FUNCTION "Ramp_down_folgen" : VOID
TITLE =
AUTHOR : 'Kleißler'
VERSION : 0.1

BEGIN
NETWORK
TITLE =Abfrage Anlage ist EIN
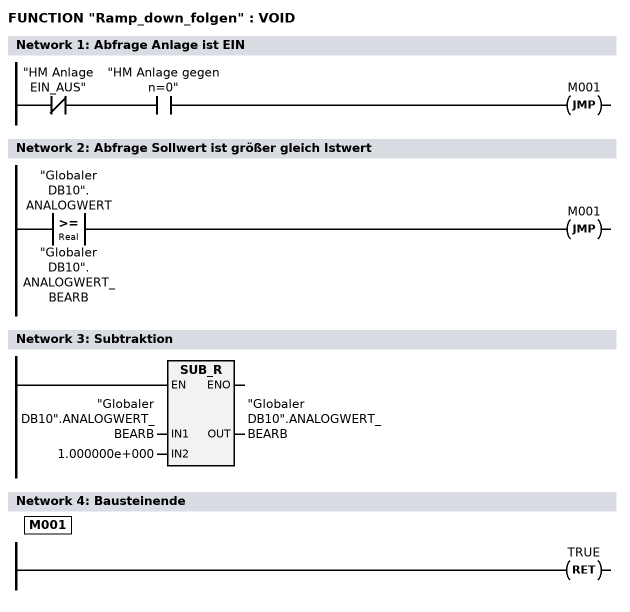
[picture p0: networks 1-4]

      UN    "HM Anlage EIN_AUS";
      U     "HM Anlage gegen n=0";
      SPB   M001;


NETWORK
TITLE =Abfrage Sollwert ist größer gleich Istwert

      L     "Globaler DB10".ANALOGWERT;
      L     "Globaler DB10".ANALOGWERT_BEARB;
      >=R   ;
      SPB   M001;




NETWORK
TITLE =Subtraktion

      L     "Globaler DB10".ANALOGWERT_BEARB;
      L     1.000000e+000;
      -R    ;
      T     "Globaler DB10".ANALOGWERT_BEARB;
      NOP   0;



NETWORK
TITLE =Bausteinende

M001: BE    ;


END_FUNCTION

FUNCTION "Analog ausgeben" : VOID
TITLE =Analogwert ausgeben
AUTHOR : 'Kleißler'
VERSION : 0.1

BEGIN
NETWORK
TITLE =Analogwert normiert (0...100) ausgeben auf PAW 820

      U     "immer low";
      =     L      0.0;
      BLD   103;
      U     "immer high";
      SPBNB _001;
      CALL "UNSCALE" (
           IN                       := "Globaler DB10".ANALOGWERT_BEARB,
           HI_LIM                   := 1.000000e+002,
           LO_LIM                   := 0.000000e+000,
           BIPOLAR                  := L      0.0,
           RET_VAL                  := "Globaler DB10".FC_106_Fehlerinfo,
           OUT                      := PAW  820);
_001: NOP   0;
END_FUNCTION

